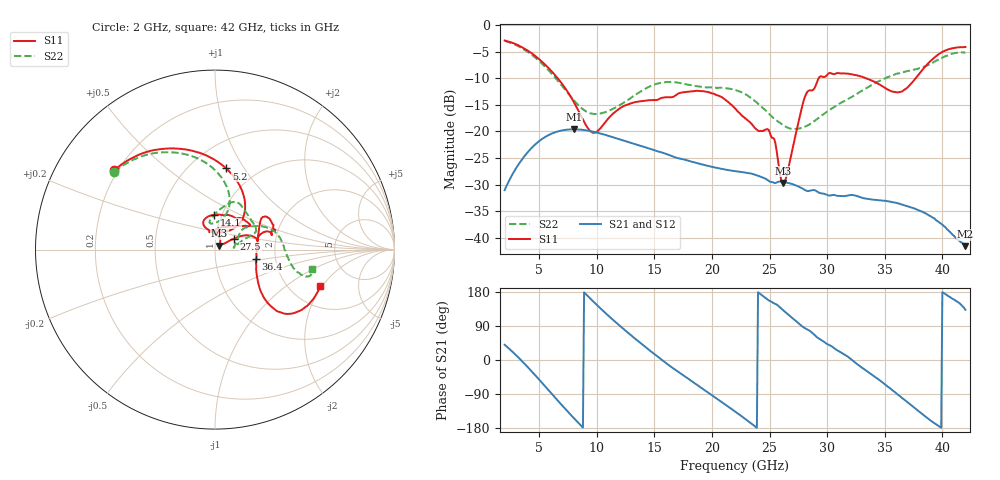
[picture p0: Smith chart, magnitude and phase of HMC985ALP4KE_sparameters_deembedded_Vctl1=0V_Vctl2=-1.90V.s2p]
!s2p File: Measurements: S11, S21, S12, S22
# GHz S dB R 50.0
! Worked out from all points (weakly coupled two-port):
!   401 points, 2 GHz to 42 GHz, reference 50 ohm
!   highest |S21| = -19.61 dB at 8 GHz (marker M1); lowest = -41.6 dB at 42 GHz (marker M2)
!   lowest |S11| = -29.7 dB at 26.2 GHz (marker M3), VSWR 1.07, Z = 52.4 + j2.37 ohm
!   |S11| at or under -10 dB: 6.6 GHz to 29.27 GHz (22.67 GHz wide, 126 % of centre); 33.36 GHz to 37.7 GHz (4.332 GHz wide, 12.2 % of centre)
!   |S22| runs from -19.6 to -3.0 dB; largest |S21 - S12| = 0.00013
!   S11 on the Smith chart (normalised r, x): 2 GHz: 0.19, +0.34; 5.2 GHz: 0.73, +0.83; 14.1 GHz: 0.92, +0.37; 27.5 GHz: 1.22, +0.15; 36.4 GHz: 1.58, -0.18; 42 GHz: 2.90, -1.91
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2  -2.91 141.7  -31.05 40.3  -31.06 40.2  -2.99 142.3
3.6  -4.30 112.5  -25.02 -5.8  -25.02 -5.8  -4.51 114.3
5.2  -6.81 82.1  -21.51 -58.6  -21.52 -58.6  -7.19 89.2
8  -14.45 46.9  -19.61 -153.0  -19.62 -153.1  -14.13 73.7
8.7  -17.38 52.1  -19.70 -175.3  -19.70 -175.3  -15.69 80.6
9.8  -20.27 86.6  -20.12 151.3  -20.12 151.3  -16.75 95.1
12.1  -15.54 113.0  -21.56 87.7  -21.57 87.7  -14.93 95.8
14.1  -14.23 91.1  -22.91 37.3  -22.92 37.3  -12.12 77.9
15.4  -13.94 73.1  -23.83 6.4  -23.83 6.4  -10.95 69.4
19.3  -12.46 34.4  -26.30 -78.2  -26.30 -78.3  -11.65 40.4
22  -15.68 52.3  -27.46 -135.7  -27.47 -135.7  -12.21 23.2
25  -20.09 98.4  -29.42 156.2  -29.43 156.2  -16.82 16.1
26.2  -29.73 43.9  -29.50 130.8  -29.51 130.8  -18.88 8.4
27.5  -18.35 30.1  -30.36 96.9  -30.36 97.0  -19.49 6.5
28.1  -13.33 20.8  -31.06 83.4  -31.08 83.3  -19.11 10.7
28.7  -12.29 12.9  -31.07 71.9  -31.05 71.8  -18.35 16.4
31  -9.06 23.3  -32.13 23.5  -32.13 23.5  -14.88 35.7
33.3  -9.94 34.3  -32.62 -25.9  -32.63 -26.0  -12.03 31.3
35.4  -12.27 12.2  -33.18 -73.4  -33.20 -73.5  -9.70 20.7
36.4  -12.58 -13.0  -33.71 -97.7  -33.69 -97.7  -8.93 14.1
39.5  -5.81 -43.4  -36.76 -170.8  -36.77 -170.8  -6.68 -14.0
42  -4.14 -19.0  -41.58 132.5  -41.53 132.6  -5.18 -11.5
